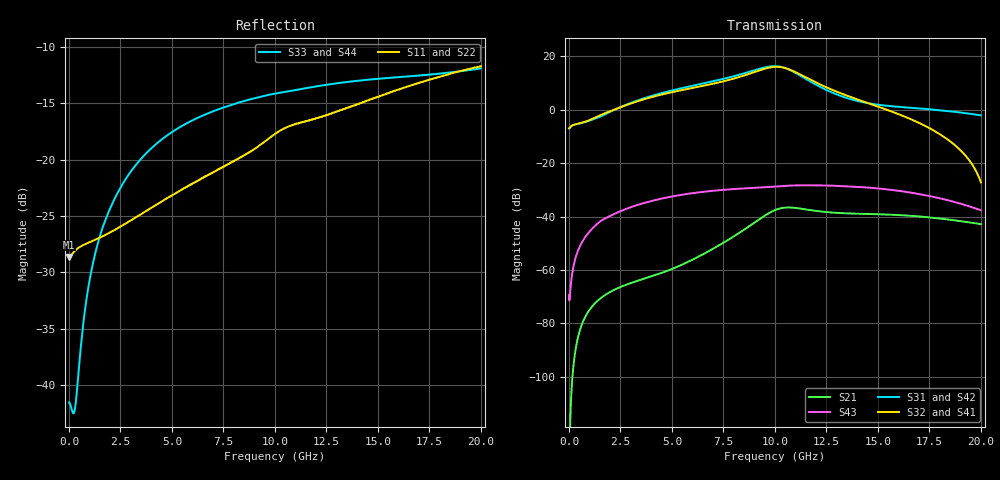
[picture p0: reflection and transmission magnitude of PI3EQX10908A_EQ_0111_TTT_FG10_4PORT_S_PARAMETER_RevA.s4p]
! NPort=4 DATA=2000 NOISE=0 GROUPDELAY=0 COMPLEX_DATAFORMAT=POLAR
! NumOfBlock=1 NumOfParam=0
! .MODEL Smodel S TSTONEFILE=PI3EQX10908A_EQ_0111_TTT_FG10_4PORT_S_PARAMETER_RevA.s4p TYPE=S
!  -- The above .MODEL line can be used for the S element in the netlist.
! The s parameter is extracted from the linear redriver, it is not bi-directional; only s(4,1)s(4,2) and s(3,1)s(3,2)
! should be the insertion loss
!Port definition:
!Port1 = input+
!Port2 = input-
!Port3 = output+
!Port4 = output-
# Hz S MA R  50
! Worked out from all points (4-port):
!   2000 points, 10 MHz to 20 GHz, reference 50 ohm
!   strongest paths, dB at 10 MHz, 5.01 GHz, 10.01 GHz, 15.01 GHz, 20 GHz:
!     S32: -6.9, 6.6, 16.1, 1.2, -27.1
!     S41: -6.9, 6.6, 16.1, 1.2, -27.0
!     S31: -6.9, 7.3, 16.3, 1.9, -2.1
!     S42: -6.9, 7.3, 16.3, 1.9, -2.1
!     S43: -69.4, -32.4, -28.7, -29.4, -37.6
!     S21: -127.2, -59.6, -37.5, -39.1, -42.8
!   lowest |S11| = -28.6 dB at 10 MHz (marker M1), VSWR 1.08, Z = 46.4 - j0.024 ohm
!   |S11| at or under -10 dB: start of sweep to end of sweep
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1e7  0.03701 -179.6  4.343e-07 14.5  0 0.0  0 0.0
     4.343e-07 14.5  0.03701 -179.6  0 0.0  0 0.0
     0.451 1.0  0.451 -179.0  0.008374 26.0  0.00034 -27.1
     0.451 -179.0  0.451 1.0  0.00034 -27.1  0.008374 26.0
7.29e9  0.09066 -118.4  0.002905 134.1  6.59e-07 57.5  3.086e-07 133.8
        0.002905 134.2  0.09069 -118.4  3.087e-07 133.8  6.591e-07 57.5
        3.638 -54.2  3.27 119.3  0.1676 7.3  0.03127 10.5
        3.271 119.3  3.638 -54.2  0.03127 10.5  0.1676 7.3
9.4e9  0.1182 -111.1  0.009814 113.5  3.226e-06 13.6  2.013e-06 117.7
       0.009817 113.6  0.1182 -111.1  2.014e-06 117.7  3.227e-06 13.6
       6.077 -111.5  5.72 63.0  0.1911 -8.7  0.03528 -10.7
       5.721 63.0  6.077 -111.5  0.03528 -10.7  0.1911 -8.7
1.044e10  0.1373 -111.7  0.01469 75.6  4.748e-06 -20.5  5.121e-06 82.1
          0.01469 75.6  0.1373 -111.7  5.124e-06 82.1  4.75e-06 -20.5
          6.17 -162.5  6.142 10.8  0.1993 -15.5  0.03757 -21.3
          6.142 10.8  6.17 -162.5  0.03757 -21.3  0.1993 -15.5
1.146e10  0.1474 -113.2  0.01373 44.0  5.125e-06 -29.5  8.095e-06 45.2
          0.01373 44.0  0.1474 -113.2  8.098e-06 45.2  5.124e-06 -29.5
          3.885 157.8  4.131 -32.6  0.207 -21.2  0.03865 -33.9
          4.131 -32.6  3.884 157.9  0.03865 -33.9  0.207 -21.2
1.362e10  0.1714 -111.6  0.01148 15.4  1.367e-05 -37.2  1.677e-05 -4.5
          0.01146 15.4  0.1715 -111.6  1.678e-05 -4.5  1.367e-05 -37.2
          1.608 129.8  1.772 -79.9  0.2215 -32.5  0.03684 -60.2
          1.771 -79.8  1.608 129.9  0.03684 -60.2  0.2215 -32.5
2e10  0.2598 -114.5  0.007264 -41.2  9.008e-05 -147.8  7.224e-05 -138.1
      0.007256 -40.9  0.2599 -114.5  7.225e-05 -138.1  9.006e-05 -147.8
      0.7879 57.1  0.04394 174.2  0.2539 -52.2  0.01316 -136.7
      0.04447 175.3  0.7889 57.1  0.01316 -136.7  0.2539 -52.2
